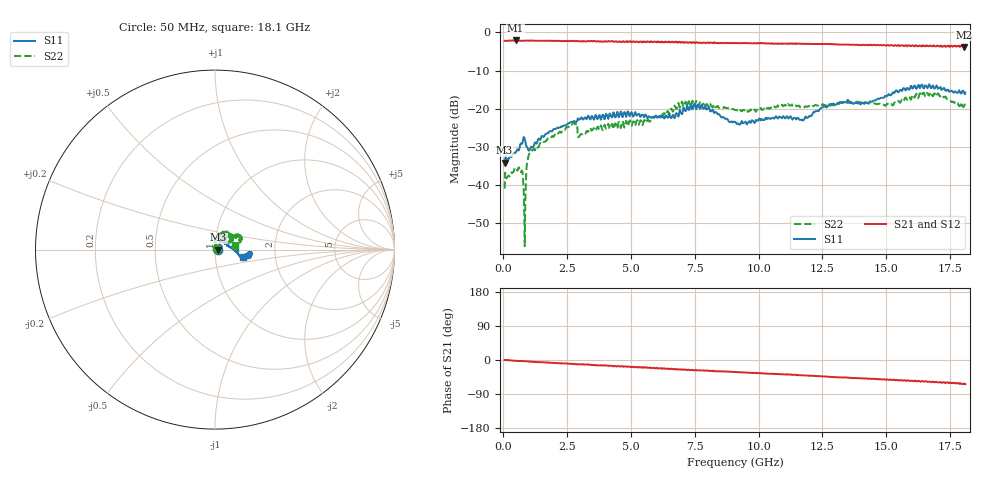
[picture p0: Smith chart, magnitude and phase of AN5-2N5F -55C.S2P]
! Network Analyzer HP8720D.06.14 Serial No. US36140669
! 12 Jan 2005  10:45:16
! Frequency  S11  S21  S12  S22
# HZ  S  DB R 50
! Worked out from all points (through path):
!   801 points, 50 MHz to 18.1 GHz, reference 50 ohm
!   highest |S21| = -2.10 dB at 478.7 MHz (marker M1); lowest = -3.8 dB at 18.03 GHz (marker M2)
!   group delay of S21, straight-line fit = 9.4 ps
!   lowest |S11| = -34.2 dB at 50 MHz (marker M3), VSWR 1.04, Z = 52 - j0.113 ohm
!   |S11| at or under -10 dB: start of sweep to end of sweep
!   |S22| runs from -56.1 to -15.7 dB; largest |S21 - S12| = 0.025
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5e7  -34.19 -3.2  -2.18 0.1  -2.17 -0.4  -40.95 20.4
4.786875e8  -31.50 31.7  -2.10 -2.0  -2.12 -2.4  -35.81 27.1
6.8175e8  -29.15 34.1  -2.18 -2.8  -2.18 -3.2  -36.68 27.3
7.945625e8  -27.47 31.8  -2.19 -3.2  -2.15 -3.3  -41.05 5.4
8.848125e8  -29.53 17.3  -2.13 -3.2  -2.13 -3.6  -38.98 127.9
9.97625e8  -31.00 27.5  -2.16 -3.8  -2.15 -4.3  -32.12 90.1
1.110438e9  -30.06 38.8  -2.17 -4.5  -2.09 -4.8  -31.29 82.4
1.742188e9  -26.46 53.1  -2.16 -6.6  -2.17 -7.1  -27.74 82.1
2.689812e9  -23.47 55.3  -2.24 -10.2  -2.24 -10.5  -24.10 84.0
3.073375e9  -22.33 55.9  -2.31 -11.8  -2.25 -12.0  -26.67 90.3
6.074188e9  -22.26 49.4  -2.47 -22.6  -2.47 -22.5  -22.24 73.0
6.931562e9  -20.70 49.8  -2.63 -25.7  -2.55 -25.4  -19.49 61.7
7.563312e9  -20.14 52.5  -2.58 -27.2  -2.73 -28.3  -18.02 39.4
9.075e9  -23.48 44.3  -2.78 -31.6  -2.72 -32.0  -20.33 29.1
1.169225e10  -22.85 18.1  -2.95 -40.5  -2.89 -40.9  -19.56 32.2
1.209838e10  -21.59 9.3  -3.00 -41.6  -2.99 -42.1  -19.41 35.4
1.284294e10  -18.85 -3.0  -3.05 -44.9  -3.02 -45.2  -18.96 35.0
1.421925e10  -18.36 -5.4  -3.28 -48.7  -3.21 -49.1  -18.48 33.5
1.509919e10  -16.18 -14.0  -3.39 -52.7  -3.25 -52.4  -19.03 34.7
1.667856e10  -13.59 -6.8  -3.60 -56.8  -3.41 -57.5  -16.56 24.2
1.803231e10  -15.55 -17.9  -3.80 -62.4  -3.80 -64.0  -19.48 18.8
1.81e10  -15.77 -15.4  -3.68 -63.7  -3.67 -64.3  -19.08 10.8
